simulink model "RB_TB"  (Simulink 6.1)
settings: Solver=ode3  SolverMode=SingleTasking  StartTime=0  StopTime=0.1  FixedStep=0.01  RelTol=1e-3
libraries: simulink x2
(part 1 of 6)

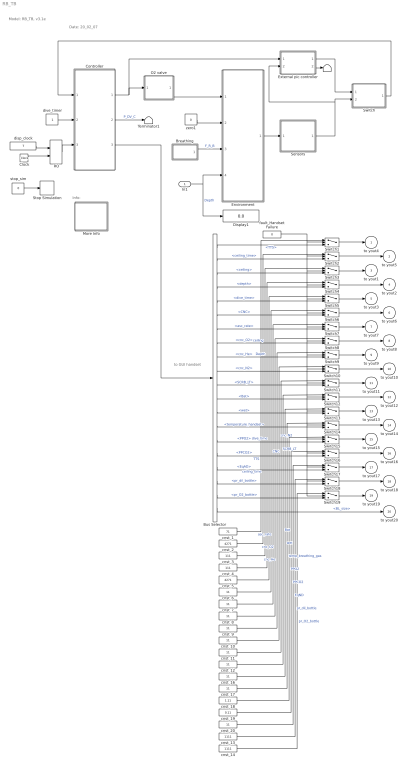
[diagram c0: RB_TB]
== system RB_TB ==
  note: Model: RB_TB, v3.1e
  note: Date: 20_02_07
  note: to GUI handset
  note: Info:
  In1 : Inport  Port=1  LatchInput=off
  Breathing : Subsystem
  Bus Selector : BusSelector  DialogController=Simulink.DDGSource_Bus  OutputSignals=TTS,ceiling_time,ceiling,depth,dive_time,CNC,asc_rate,cnc_O2,cnc_He,cnc_N2,SCRB_LT,Bat,wet,temperature_handset,PPO2,PPCO2,EqAD,pr_dil_bottle,pr_O2_bottle,BL_size
  Clock : Clock
  Controller : Subsystem
  Display1 : Display
  Environment : Subsystem
  External pic controller : Subsystem
  More Info : Subsystem
  O2 valve : Subsystem
  RO : RelationalOperator  Operator===  LogicOutDataTypeMode=Boolean
  Sensors : Subsystem
  Stop Simulation : Stop
  Switch : Subsystem
  Switch{1..19} (19 alike) : Switch  Threshold=0.5
  T : Terminator
  Terminator1 : Terminator
  cnst_1 : Constant  Value=71
  cnst_{6..12,16..17,20} (10 alike) : Constant  Value=11
  cnst_13 : Constant  Value=1111
  cnst_14 : Constant  Value=1111
  cnst_18 : Constant  Value=1.11
  cnst_19 : Constant  Value=0.11
  cnst_2 : Constant  Value=4271
  cnst_3 : Constant  Value=111
  cnst_4 : Constant  Value=111
  cnst_5 : Constant  Value=4271
  disp_clock : Constant  Value=7
  dive_timer : Constant
  fault_Handset Failure : Constant  Value=0
  stop_sim : Constant  Value=0
  zero1 : Constant  Value=0
  to yout4 : Outport
  to yout5 : Outport  Port=2
  to yout1 : Outport  Port=3
  to yout2 : Outport  Port=4
  to yout3 : Outport  Port=5
  to yout6 : Outport  Port=6
  to yout7 : Outport  Port=7
  to yout8 : Outport  Port=8
  to yout9 : Outport  Port=9
  to yout10 : Outport  Port=10
  to yout11 : Outport  Port=11
  to yout12 : Outport  Port=12
  to yout13 : Outport  Port=13
  to yout14 : Outport  Port=14
  to yout15 : Outport  Port=15
  to yout16 : Outport  Port=16
  to yout17 : Outport  Port=17
  to yout18 : Outport  Port=18
  to yout19 : Outport  Port=19
  to yout20 : Outport  Port=20
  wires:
  Controller/1(O2 control) -> O2 valve/1(IN), External pic controller/1(valve_in)
  Breathing/1(Metabolic) -> Environment/3(Metablic)  "F_R_B"
  Environment/1(bus) -> Sensors/1(In)
  disp_clock/1 -> RO/1
  Clock/1 -> RO/2
  RO/1 -> Controller/3(disp_clock)
  External pic controller/1(sensor_out) -> Switch/1(In1)
  Sensors/1(Out) -> Switch/2(In2), External pic controller/2(sensor_in)
  Switch/1(Out) -> Controller/1(InBus)
  Controller/2(Dil valve) -> Terminator1/1  "P_DV_C"
  zero1/1 -> Environment/2(Dil valve)
  O2 valve/1(Orf_size) -> Environment/1(Orf_size)
  dive_timer/1 -> Controller/2(dive_timer)
  cnst_1/1 -> Switch1/1  "TTS"
  cnst_2/1 -> Switch2/1  "ceiling_time"
  cnst_4/1 -> Switch4/1  "Depth"
  cnst_5/1 -> Switch5/1  "dive_time"
  cnst_6/1 -> Switch6/1  "CNC"
  cnst_7/1 -> Switch7/1  "asc_rate"
  cnst_8/1 -> Switch8/1  "cnc_O2"
  cnst_9/1 -> Switch9/1  "cnc_He"
  cnst_10/1 -> Switch10/1  "cnc_N2"
  cnst_11/1 -> Switch11/1  "SCRB_LT"
  cnst_12/1 -> Switch12/1  "Bat"
  cnst_16/1 -> Switch13/1  "wet"
  cnst_17/1 -> Switch14/1  "temp_breathing_gas"
  cnst_18/1 -> Switch15/1  "PPO2"
  cnst_19/1 -> Switch16/1  "PPCO2"
  cnst_20/1 -> Switch17/1  "EqND"
  cnst_13/1 -> Switch18/1  "pr_dil_bottle"
  cnst_14/1 -> Switch19/1  "pr_O2_bottle"
  Controller/3(bus) -> Bus Selector/1
  Bus Selector/1 -> Switch1/3  "<TTS>"
  Bus Selector/2 -> Switch2/3  "<ceiling_time>"
  Bus Selector/3 -> Switch3/3  "<ceiling>"
  Bus Selector/4 -> Switch4/3  "<depth>"
  Bus Selector/5 -> Switch5/3  "<dive_time>"
  Bus Selector/6 -> Switch6/3  "<CNC>"
  Bus Selector/7 -> Switch7/3  "<asc_rate>"
  Bus Selector/8 -> Switch8/3  "<cnc_O2>"
  Bus Selector/9 -> Switch9/3  "<cnc_He>"
  Bus Selector/10 -> Switch10/3  "<cnc_N2>"
  Bus Selector/11 -> Switch11/3  "<SCRB_LT>"
  Bus Selector/12 -> Switch12/3  "<Bat>"
  Bus Selector/13 -> Switch13/3  "<wet>"
  Bus Selector/14 -> Switch14/3  "<temperature_handset>"
  Bus Selector/15 -> Switch15/3  "<PPO2>"
  Bus Selector/16 -> Switch16/3  "<PPCO2>"
  Bus Selector/17 -> Switch17/3  "<EqAD>"
  Bus Selector/18 -> Switch18/3  "<pr_dil_bottle>"
  Bus Selector/19 -> Switch19/3  "<pr_O2_bottle>"
  Switch19/1 -> to yout19/1
  Switch18/1 -> to yout18/1
  Switch17/1 -> to yout17/1
  Switch16/1 -> to yout16/1
  Switch15/1 -> to yout15/1
  Switch14/1 -> to yout14/1
  Switch13/1 -> to yout13/1
  Switch12/1 -> to yout12/1
  Switch11/1 -> to yout11/1
  Switch10/1 -> to yout10/1
  Switch9/1 -> to yout9/1
  Switch8/1 -> to yout8/1
  Switch7/1 -> to yout7/1
  Switch6/1 -> to yout6/1
  Switch5/1 -> to yout3/1
  Switch4/1 -> to yout2/1
  Switch3/1 -> to yout1/1
  Switch2/1 -> to yout5/1
  Switch1/1 -> to yout4/1
  fault_Handset Failure/1 -> Switch18/2, Switch19/2, Switch17/2, Switch16/2, Switch15/2, Switch14/2, Switch13/2, Switch12/2, Switch11/2, Switch10/2, Switch9/2, Switch8/2, Switch7/2, Switch6/2, Switch5/2, Switch4/2, Switch3/2, Switch2/2, Switch1/2
  In1/1 -> Display1/1, Environment/4(Depth)  "Depth"
  External pic controller/2(valve_out) -> T/1
  cnst_3/1 -> Switch3/1  "ceiling"
  stop_sim/1 -> Stop Simulation/1
  Bus Selector/20 -> to yout20/1  "<BL_size>"

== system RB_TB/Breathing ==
  note: Model: RB_TB/Breathing
  rate_metabolic : Sin  Amplitude=0.015  Bias=0.015  Frequency=1.4661  SampleTime=0
  Metabolic : Outport
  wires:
  rate_metabolic/1 -> Metabolic/1

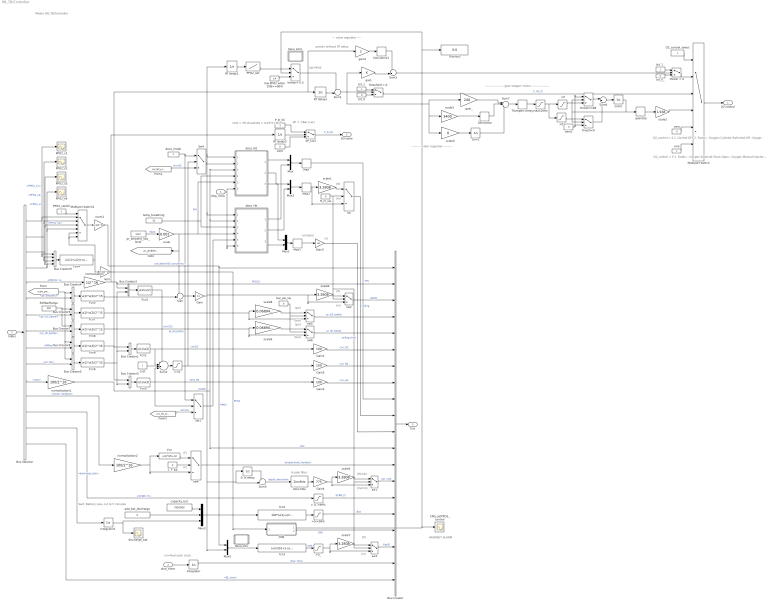
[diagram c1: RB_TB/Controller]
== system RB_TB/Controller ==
  note: Model: RB_TB/Controller
  note: dP = -1Bar (var)
  note: CO2 = 3% threshold = 0.03*2^16
  note: (minute)
  note: (s)
  note: ini=final each clock
  note: Fault: Battery Low, cut to 5 minutes
  note: predicr without RT delay
  note: O2_control = 4 1. Control OFF 2. Faults: - Oxygen Cylinder Switched Off - Oxygen First Stage Failure - Oxygen Solenoid Stuck Closed
  note: O2_control = 5 1. Faults: - Oxygen Solenoid Stuck Open - Oxygen Manual Injector Failure
  note: 6-pole filter
  note: ------------------- gear stepper motor ------------------
  note: Set PPO2
  note: --------- motor regulator ---------
  note: --- valve regulator ----
  note: (m)
  note: (ft)
  note: (ft)
  note: (m)
  note: (ft/min)
  note: (m/min)
  note: (m)
  note: (ft)
  note: (C)
  note: (F)
  note: (psi)
  note: (bar)
  note: (psi)
  note: (bar)
  note: HANDSET ALARM
  InBus : Inport  Port=1  LatchInput=off
  dive_timer : Inport  Port=2  LatchInput=off
  disp_clock : Inport  Port=3  LatchInput=off
  0.1s delay : UnitDelay  SampleTime=0.1
  300barRange : Constant  Value=300
  <0 : Saturate  UpperLimit=0  LowerLimit=-inf
  "> 0, <99%" : Saturate  UpperLimit=99  LowerLimit=0
  >0 : Saturate  UpperLimit=inf  LowerLimit=0
  >0,<99% : Saturate  UpperLimit=99  LowerLimit=0
  >0_ : Saturate  UpperLimit=inf  LowerLimit=0
  >=0 : Saturate  UpperLimit=inf  LowerLimit=0
  Bus Creator : BusCreator  DialogController=Simulink.DDGSource_Bus  Inputs=20
  Bus Creator{1..8} (8 alike) : BusCreator  DialogController=Simulink.DDGSource_Bus  Inputs=2
  Bus Creator9 : BusCreator  DialogController=Simulink.DDGSource_Bus
  Bus Selector : BusSelector  DialogController=Simulink.DDGSource_Bus  OutputSignals=PPO2_s1,PPO2_s2,PPO2_s3,PPO2_s4,PPCO2_s,pr_ambient,pr_O2_bottle,pr_dil_bottle,PPHe,pr_BL,wet,temp_handset,SCRB_LT,discharge_bat,BL_size
  CNS : Subsystem
  CNS_setPPO2_control : Scope
  C_F_sw : Constant  Value=0
  Derivative : Derivative
  Derivative1 : Derivative
  Display2 : Display
  Fcn : Fcn  Expr=u(1)*9/5+32
  Fcn1 : Fcn  Expr=u(1)/u(2)
  Fcn2 : Fcn  Expr=u(1)/u(2)
  Fcn3 : Fcn  Expr=u(1)/u(2)
  Fcn4 : Fcn  Expr=(u(1)+u(2)+u(3)+u(4))/4
  Fcn{5..8} (4 alike) : Fcn  Expr=u(1)*u(2)/2^15
  Fcn9 : Fcn  Expr=u(1)*u(2)/2^16
  Gain : Gain  Gain=10
  Gain1 : Gain  Gain=100
  Gain2 : Gain  Gain=100
  Gain3 : Gain  Gain=60
  Gain4 : Gain  Gain=775
  Gain5 : Gain  Gain=100
  Integrator : Integrator
  Integrator1 : Integrator
  Max : MinMax  Function=max
  Max1 : MinMax  Function=max
  Max2 : MinMax  Function=max
  More Info : Subsystem
  More Info1 : Subsystem
  Multiport Switch : MultiPortSwitch  Inputs=5
  Multiport Switch1 : MultiPortSwitch  Inputs=6
  Mux{,1..2,5} (4 alike) : Mux  Inputs=2
  Mux3 : Mux  Inputs=3
  O2_control_select : Constant
  PPO2_s{1..4} (4 alike) : Scope
  PPO2_set : Lookup  DialogController=Simulink.DDGSource  InputValues="[0         4.3001           1000]"  OutputValues="[0.7      1.0001      1.0002]"  LookUpMeth=Interpolation-Use End Values
  PPO2_switch : Constant
  P_D_VC : Constant  Value=-1
  RT delay1 : UnitDelay  SampleTime=0.1
  RT delay2 : UnitDelay  SampleTime=0.1
  RT delay3 : UnitDelay  SampleTime=0.1
  SP_CO2 : Switch  Threshold=0.03
  Sum : Sum  Inputs=-+|
  Sum1 : Sum  Inputs=+-|
  Sum2 : Sum  Inputs=--+-|
  Sum3 : Sum  Inputs=-+|
  Sum4 : Sum  Inputs=|++
  Sum5 : Sum  Inputs=-+|
  Sum7 : Sum  Inputs=|+++
  Sw1 : MultiPortSwitch  Inputs=2
  Sw4 : MultiPortSwitch  Inputs=2
  Transport Delay : TransportDelay  DelayTime=0.01
  Zero : Constant  Value=0
  Zero-Pole : ZeroPole  Zeros=[0]  Poles=[-1 -1 -1 -1 -1 -1]
  add_bat_discharge : Constant  Value=0
  bar_psi_sw : Constant  Value=0
  bit_0 : Constant  Value=0
  bit_0_ : Constant  Value=0
  bit_1 : Constant
  bit_1_ : Constant
  capacity_bat : Constant  Value=7920000
  cnst : Constant
  deco_He : Subsystem
  deco_N2 : Subsystem
  deco_mode : Constant
  discharge_bat : Scope
  fcn2 : Fcn  Expr=100*(u(1)-u(2)-u(3))/u(1)
  fcn3 : Fcn  Expr=(u(2)/10+1-u(1))/0.79-1
  ft_m_sw : Constant  Value=0
  gain : Gain
  gain1 : Gain  Gain=2
  gain_ : Gain  Gain=240
  low PPO2 when CNS>=90% : Constant  Value=0.4
  max100Hz : Saturate  UpperLimit=100  LowerLimit=-100
  norm : Gain  Gain=2.3/2^16
  norm1 : Gain  Gain=2.3/2^16
  normalisation : Gain  Gain=1/2^16
  normalisation1 : Gain  Gain=100/2^16
  normalisation2 : Gain  Gain=100/2^16
  one : Constant
  pr_ambient_sea_level : Constant  Value=1010
  quantize : Quantizer  QuantizationInterval=1
  scale : Gain  Gain=0.001
  scale{1,5..7} (4 alike) : Gain  Gain=3.2808
  scale2 : Gain  Gain=1/168
  scale3 : Gain  Gain=3400
  scale4 : Gain  Gain=0
  scale8 : Gain  Gain=0.0689476
  scale9 : Gain  Gain=0.0689476
  sum1 : Integrator
  sum2 : Integrator
  sw{,1..6} (7 alike) : Switch  Threshold=0.5
  temp_breathing : Constant  Value=33
  thresh = 0 : Switch  Criteria=u2 > Threshold
  thresh= 0.5 : Switch  Threshold=0.5
  thresh=0 : Switch
  thresh=168 : Switch  Threshold=168
  threshold = 0 : Switch  Criteria=u2 > Threshold
  zero : Constant  Value=0
  zero1 : Constant  Value=0
  O2 control : Outport
  Dil valve : Outport  Port=2
  bus : Outport  Port=3
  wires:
  RT delay2/1 -> Sum1/2
  bit_1/1 -> threshold = 0/1
  bit_0/1 -> threshold = 0/3
  temp_breathing/1 -> deco_N2/4(Temp_air), deco_He/3(Temp_air)
  deco_N2/1(TTS_N2) -> Mux/1
  deco_He/1(TTS_He) -> Mux/2
  Mux/1 -> Max/1
  Mux1/1 -> Max1/1
  deco_He/3(ceiling_time_He) -> Mux1/2
  deco_N2/3(ceiling_time_N2) -> Mux1/1
  Mux2/1 -> Max2/1
  deco_N2/2(ceiling_N2) -> Mux2/1
  deco_He/2(ceiling_He) -> Mux2/2
  Max/1 -> Bus Creator/9  "TTS"
  pr_ambient_sea_level/1 -> scale/1  "mbar"
  Bus Creator/1 -> bus/1
  InBus/1 -> Bus Selector/1
  Bus Selector/3 -> Bus Creator9/3, Multiport Switch1/4, PPO2_s3/1  "<PPO2_s3>"
  Bus Selector/4 -> Bus Creator9/4, Multiport Switch1/5, PPO2_s4/1  "<PPO2_s4>"
  norm/1 -> CNS/1(PPO2), RT delay2/1, gain1/1, Bus Creator1/1  "PPO2"
  normalisation/1 -> RT delay3/1, Bus Creator2/1, Bus Creator/2  "PPCO2"
  Sum/1 -> Gain/1
  Gain/1 -> 0.1s delay/1, Sum5/2, Mux5/2, deco_He/1(depth), deco_N2/1(depth), RT delay1/1, scale6/1, sw2/3  "Depth"
  Gain5/1 -> Bus Creator/7  "cnc_N2"
  Fcn3/1 -> Sum2/4, Sw1/2, Gain2/1  "sens He"
  disp_clock/1 -> deco_N2/6(disp_clock), deco_He/6(disp_clock)
  Integrator/1 -> Bus Creator/19  "dive_time"
  >0,<99%/1 -> Bus Creator/16  "Bat"
  RT delay3/1 -> SP_CO2/2
  P_D_VC/1 -> SP_CO2/1
  SP_CO2/1 -> Dil valve/1  "P_D_VC"
  Zero/1 -> SP_CO2/3
  Bus Selector/5 -> normalisation/1  "<PPCO2_s>"
  scale/1 -> deco_He/4(P_amb_sea_level), deco_N2/5(P_amb_sea_level), [pr_ambient_sea_level], Sum/1  "bar"
  Max1/1 -> Gain3/1
  Gain3/1 -> Bus Creator/11  "ceiling_time"
  Mux3/1 -> fcn2/1
  fcn2/1 -> >0,<99%/1
  Fcn1/1 -> Sum2/2, Gain1/1  "cncO2"
  Gain1/1 -> Bus Creator/6  "cnc_O2"
  Gain2/1 -> Bus Creator/8  "cnc_He"
  Bus Creator2/1 -> Fcn2/1
  cnst/1 -> Sum2/3
  Fcn2/1 -> Sum2/1  "cncCO2"
  deco_mode/1 -> Sw4/1, Sw1/1
  [cnc_N2_presize] -> Sw4/3  "sim N2"
  [cnc_He_presize] -> Sw1/3  "sim He"
  Sw4/1 -> deco_N2/2(cnc_N2)
  Sw1/1 -> deco_He/5(cnc_He)
  Mux5/1 -> fcn3/1
  fcn3/1 -> >0_/1  "CNS"
  CNS/2(CNS) -> Bus Creator/17  "CNC"
  dive_timer/1 -> Integrator/1
  capacity_bat/1 -> Mux3/1
  add_bat_discharge/1 -> Mux3/2
  Integrator1/1 -> discharge_bat/1, Mux3/3
  Bus Selector/2 -> Bus Creator9/2, Multiport Switch1/3, PPO2_s2/1  "<PPO2_s2>"
  Bus Selector/1 -> Multiport Switch1/2, Bus Creator9/1, PPO2_s1/1  "<PPO2_s1>"
  Sum1/1 -> gain/1, threshold = 0/2, gain_/1, scale4/1, scale3/1
  gain1/1 -> Derivative1/1
  O2_control_select/1 -> Multiport Switch/1
  Multiport Switch/1 -> O2 control/1
  bit_1_/1 -> thresh = 0/1
  bit_0_/1 -> thresh = 0/3
  Sum3/1 -> thresh = 0/2
  thresh = 0/1 -> Multiport Switch/2
  threshold = 0/1 -> Multiport Switch/3  "F_O2_O"
  "> 0, <99%"/1 -> Bus Creator/15  "SCRB_LT"
  Bus Selector/14 -> Integrator1/1  "<discharge_bat>"
  Bus Selector/13 -> "> 0, <99%"/1  "<SCRB_LT>"
  Bus Selector/11 -> normalisation1/1  "<wet>"
  normalisation1/1 -> deco_He/2(Wet), deco_N2/3(Wet), Bus Creator/12  "wet"
  Bus Selector/12 -> normalisation2/1  "<temp_handset>"
  [scale_pressure] -> Bus Creator4/1, Bus Creator5/1, Bus Creator8/1
  Bus Selector/6 -> Bus Creator4/2  "<pr_ambient>"
  Bus Creator4/1 -> Fcn5/1
  Fcn5/1 -> Sum/2
  Sum2/1 -> >=0/1
  >=0/1 -> Sw4/2, Gain5/1  "calculated N2 concentration"
  one/1 -> Multiport Switch/6
  Bus Creator3/1 -> Fcn3/1
  Bus Creator1/1 -> Fcn1/1
  Bus Creator5/1 -> Fcn6/1
  Bus Selector/10 -> Bus Creator5/2  "<pr_BL>"
  Fcn6/1 -> Bus Creator3/2, Bus Creator1/2, Bus Creator2/2
  Sum5/1 -> Zero-Pole/1  "depth_derivative"
  0.1s delay/1 -> Sum5/1
  Zero-Pole/1 -> Gain4/1
  Bus Selector/7 -> Bus Creator6/2  "<pr_O2_bottle>"
  Bus Creator6/1 -> Fcn7/1
  300barRange/1 -> Bus Creator6/1, Bus Creator7/1
  Bus Creator7/1 -> Fcn8/1
  Bus Selector/8 -> Bus Creator7/2  "<pr_dil_bottle>"
  Bus Creator8/1 -> Fcn9/1
  Bus Selector/9 -> Bus Creator8/2  "<PPHe>"
  Fcn9/1 -> Bus Creator3/1
  max100Hz/1 -> >0/1, <0/1
  Transport Delay/1 -> max100Hz/1
  scale3/1 -> Derivative/1
  scale4/1 -> sum1/1
  gain/1 -> Sum3/2
  Derivative1/1 -> Sum3/1
  scale2/1 -> Multiport Switch/4
  sum1/1 -> Sum7/3
  Max2/1 -> scale1/1, sw/3
  scale1/1 -> sw/1
  ft_m_sw/1 -> sw/2, sw2/2, sw1/2, sw3/2
  sw/1 -> Bus Creator/10  "ceiling"
  scale5/1 -> sw1/1
  sw1/1 -> Bus Creator/14  "asc_rate"
  Gain4/1 -> sw1/3, scale5/1
  scale6/1 -> sw2/1
  sw2/1 -> Bus Creator/3  "depth"
  sw3/1 -> Bus Creator/18  "EqAD"
  scale7/1 -> sw3/1
  >0_/1 -> sw3/3, scale7/1
  Fcn/1 -> sw4/1
  C_F_sw/1 -> sw4/2
  sw4/1 -> Bus Creator/13  "temperature_handset"
  normalisation2/1 -> sw4/3, Fcn/1
  Fcn7/1 -> scale8/1, sw5/3
  bar_psi_sw/1 -> sw5/2, sw6/2
  scale8/1 -> sw5/1
  sw5/1 -> Bus Creator/4  "pr_O2_bottle"
  Fcn8/1 -> sw6/3, scale9/1  "pr_dil_bottle"
  scale9/1 -> sw6/1
  sw6/1 -> Bus Creator/5  "pr_dil_bottle"
  PPO2_switch/1 -> Multiport Switch1/1
  RT delay1/1 -> PPO2_set/1
  low PPO2 when CNS>=90%/1 -> thresh= 0.5/3
  CNS/1(PPO2_set_Control) -> CNS_setPPO2_control/1, thresh= 0.5/2, Display2/1
  >0/1 -> thresh=168/3
  <0/1 -> thresh=0/1
  quantize/1 -> scale2/1
  zero/1 -> Multiport Switch/5
  Multiport Switch1/1 -> norm1/1
  norm1/1 -> Bus Creator/1, Mux5/1  "PPO2"
  Bus Creator9/1 -> Fcn4/1
  Fcn4/1 -> norm/1, Multiport Switch1/6, Multiport Switch1/7
  Derivative/1 -> Sum7/2
  Sum7/1 -> Transport Delay/1
  gain_/1 -> Sum7/1
  sum2/1 -> quantize/1, thresh=168/2, thresh=0/2
  thresh=168/1 -> Sum4/1
  Sum4/1 -> sum2/1
  thresh=0/1 -> Sum4/2
  zero1/1 -> thresh=0/3, thresh=168/1
  Bus Selector/15 -> Bus Creator/20  "<BL_size>"
  PPO2_set/1 -> thresh= 0.5/1
  thresh= 0.5/1 -> Sum1/1

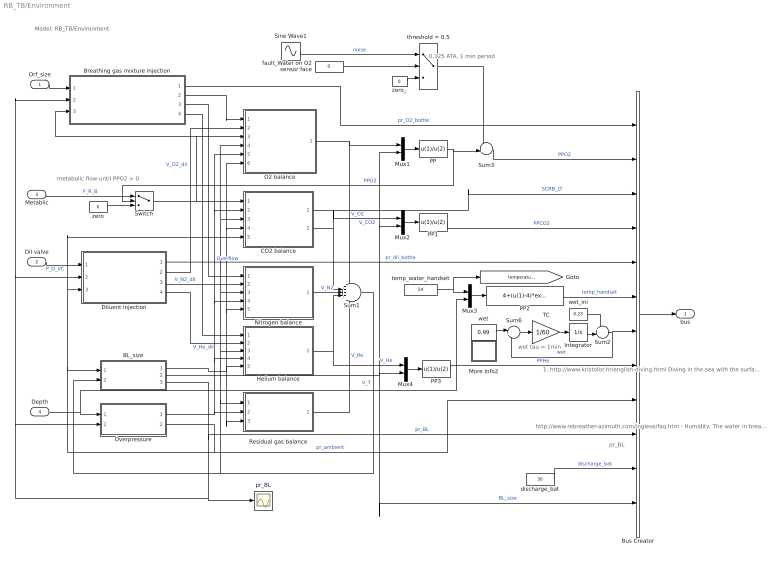
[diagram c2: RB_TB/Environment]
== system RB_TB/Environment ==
  note: Model: RB_TB/Environment
  note: metabolic flow until PPO2 > 0
  note: 0.125 ATA, 1 min period
  note: 1. http://www.kristofor.hr/english-diving.html Diving in the sea with the surface sea temperature 9 - 12 deg.C in winter, 24 - 28 degC in summer, On 20 m sea depth temperature is permanent, around 14 deg.C temperature = 14+(u(1)-14)*exp(-u(2)/7) 2. Al: Temperature goes from whatever the surface is, to 4C at 200m, and stays there below 200m. temperature = 4+(u(1)-4)*exp(-u(2)/35)
  note: http://www.rebreather-azimuth.com/inglese/faq.htm - Humidity: The water in breathing and from the chemical reaction maintain the humidity constantly at 100% in in semiclosed rebreather. The situation in open circuit is different, the gas mixture is completely dry, and the diver loses a big quantity of liquids during the dive.
  note: wet tau = 1min
  note: pr_BL
  Orf_size : Inport  Port=1  LatchInput=off
  Dil valve : Inport  Port=2  LatchInput=off
  Metablic : Inport  Port=3  LatchInput=off
  Depth : Inport  Port=4  LatchInput=off
  BL_size : Subsystem
  Breathing gas mixture injection : Subsystem
  Bus Creator : BusCreator  DialogController=Simulink.DDGSource_Bus  Inputs=12
  CO2 balance : Subsystem
  Diluent injection : Subsystem
  Helium balance : Subsystem
  Integrator : Integrator
  More Info2 : Subsystem
  Mux{1..4} (4 alike) : Mux  Inputs=2
  Nitrogen balance : Subsystem
  O2 balance : Subsystem
  Overpressure : Subsystem
  PP : Fcn  Tag=ee  Priority=306454640  Expr=u(1)/u(2)
  PP1 : Fcn  Tag=ee  Priority=306454640  Expr=u(1)/u(2)
  PP2 : Fcn  Tag=ee  Priority=306454640  Expr=4+(u(1)-4)*exp(-u(2)/35)
  PP3 : Fcn  Tag=ee  Priority=306454640  Expr=u(1)/u(2)
  Residual gas balance : Subsystem
  Sine Wave1 : Sin  Amplitude=0.125  Frequency=pi/30  SampleTime=0
  Sum1 : Sum  Inputs=+++++
  Sum2 : Sum  Inputs=++|
  Sum3 : Sum  Inputs=++|
  Sum6 : Sum  Inputs=|+-
  Switch : Switch  Criteria=u2 > Threshold
  TC : Gain  Gain=1/60
  discharge_bat : Constant  Value=30
  fault_Water on O2 sensor face : Constant  Value=0
  pr_BL : Scope
  temp_water_handset : Constant  Value=24
  threshold = 0.5 : Switch  Criteria=u2 > Threshold  Threshold=0.5
  wet : Constant  Value=0.99
  wet_ini : Constant  Value=0.23
  zero : Constant  Value=0
  zero_ : Constant  Value=0
  bus : Outport
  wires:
  Diluent injection/3(N2) -> Nitrogen balance/2(V_N2_dil)  "V_N2_dil"
  O2 balance/1(O2 in BL) -> Sum1/1, Mux1/1  "V_O2"
  Overpressure/1(Overflow) -> CO2 balance/2(Overflow), O2 balance/5(Overflow), Nitrogen balance/4(Overflow), Helium balance/4(Overflow), Residual gas balance/2(Overflow)  "Overflow"
  Sum1/1 -> Helium balance/3(gas_total), Nitrogen balance/3(gas_total), CO2 balance/3(gas_total), O2 balance/4(gas_total), Residual gas balance/1(gas_total), BL_size/2(vol_gas_total)  "V_T"
  Nitrogen balance/1(N2 in BL) -> Sum1/3  "V_N2"
  CO2 balance/2(CO2 in BL) -> Sum1/2, Mux2/1  "V_CO2"
  Dil valve/1 -> Diluent injection/1(Valve_ON/OFF)  "P_D_VC"
  Helium balance/1(He in BL) -> Mux4/1, Sum1/4  "V_He"
  Diluent injection/4(He) -> Helium balance/2(V_He_dil)  "V_He_dil"
  Residual gas balance/1(Re in BL) -> Sum1/5  "V_Re"
  PP/1 -> Sum3/2, Switch/2  "PPO2"
  Bus Creator/1 -> bus/1
  PP1/1 -> Bus Creator/4  "PPCO2"
  PP3/1 -> Bus Creator/8  "PPHe"
  BL_size/2(BL_size) -> Mux4/2, Mux2/2, Mux1/2, Bus Creator/12  "BL_size"
  Mux1/1 -> PP/1
  Mux2/1 -> PP1/1
  Mux4/1 -> PP3/1
  Orf_size/1 -> Breathing gas mixture injection/1(Orf_size)
  Breathing gas mixture injection/1(pr_breathing_mixture_bottle) -> Bus Creator/1  "pr_O2_bottle"
  Overpressure/2(pr_ambient) -> Bus Creator/9, BL_size/1(pr_ambient), Diluent injection/3(pr_ambient), CO2 balance/5(pr_ambient)  "pr_ambient"
  Diluent injection/1(pr_dil_bottle) -> Bus Creator/5  "pr_dil_bottle"
  BL_size/3(pr_BL) -> Overpressure/2(pr_BL), Breathing gas mixture injection/2(pr_BL), Diluent injection/2(pr_BL), pr_BL/1, Bus Creator/10  "pr_BL"
  Depth/1 -> Overpressure/1(Depth), Mux3/2
  Switch/1 -> CO2 balance/1(Metabolic), O2 balance/3(Metabolic), Breathing gas mixture injection/3(Metabolic)
  Metablic/1 -> Switch/1  "F_R_B"
  zero/1 -> Switch/3
  CO2 balance/1(SCRB) -> Bus Creator/3  "SCRB_LT"
  discharge_bat/1 -> Bus Creator/11  "discharge_bat"
  fault_Water on O2 sensor face/1 -> threshold = 0.5/2
  Sine Wave1/1 -> threshold = 0.5/1  "noise"
  zero_/1 -> threshold = 0.5/3
  Sum3/1 -> Bus Creator/2  "PPO2"
  threshold = 0.5/1 -> Sum3/1
  temp_water_handset/1 -> Mux3/1, [temperature_sea_level]
  Mux3/1 -> PP2/1
  PP2/1 -> Bus Creator/6  "temp_handset"
  TC/1 -> Integrator/1
  Integrator/1 -> Sum2/2
  wet_ini/1 -> Sum2/1
  Sum2/1 -> Sum6/2, Bus Creator/7  "wet"
  Sum6/1 -> TC/1
  wet/1 -> Sum6/1
  Diluent injection/2(O2) -> O2 balance/2(V_O2_dil)  "V_O2_dil"
  Breathing gas mixture injection/2(V_O2_breathing_mixture_bottle) -> O2 balance/1(V_O2_breathing)
  Breathing gas mixture injection/3(V_N2_breathing_mixture_bottle) -> Nitrogen balance/1(V_N2_breathing)
  Breathing gas mixture injection/4(V_He_breathing_mixture_bottle) -> Helium balance/1(V_He_breathing)
  BL_size/1(BL_size_ini) -> Helium balance/5(BL_size_ini), Residual gas balance/3(BL_size_ini), Nitrogen balance/5(BL_size_ini), CO2 balance/4(BL_size_ini), O2 balance/6(BL_size_ini)

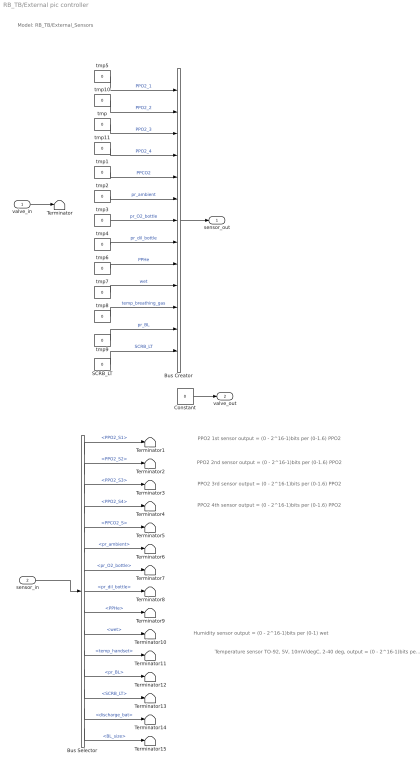
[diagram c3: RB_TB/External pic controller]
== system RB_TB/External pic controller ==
  note: Model: RB_TB/External_Sensors
  note: Humidity sensor output = (0 - 2^16-1)bits per (0-1) wet
  note: PPO2 1st sensor output = (0 - 2^16-1)bits per (0-1.6) PPO2
  note: PPO2 2nd sensor output = (0 - 2^16-1)bits per (0-1.6) PPO2
  note: PPO2 3rd sensor output = (0 - 2^16-1)bits per (0-1.6) PPO2
  note: PPO2 4th sensor output = (0 - 2^16-1)bits per (0-1.6) PPO2
  note: Temperature sensor TO-92, 5V, 10mV/degC, 2-40 deg, output = (0 - 2^16-1)bits per (0-1) wet
  valve_in : Inport  Port=1  LatchInput=off
  sensor_in : Inport  Port=2  LatchInput=off
  Bus Creator : BusCreator  DialogController=Simulink.DDGSource_Bus  Inputs=13
  Bus Selector : BusSelector  DialogController=Simulink.DDGSource_Bus  OutputSignals=PPO2_S1,PPO2_S2,PPO2_S3,PPO2_S4,PPCO2_S,pr_ambient,pr_O2_bottle,pr_dil_bottle,PPHe,wet,temp_handset,pr_BL,SCRB_LT,discharge_bat,BL_size
  Constant : Constant  Value=0
  SCRB_LT : Constant  Value=0
  Terminator{,1..15} (16 alike) : Terminator
  tmp{,1..11} (12 alike) : Constant  Value=0
  sensor_out : Outport
  valve_out : Outport  Port=2
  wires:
  tmp7/1 -> Bus Creator/10  "wet"
  tmp8/1 -> Bus Creator/11  "temp_breathing_gas"
  tmp6/1 -> Bus Creator/9  "PPHe"
  tmp4/1 -> Bus Creator/8  "pr_dil_bottle"
  tmp3/1 -> Bus Creator/7  "pr_O2_bottle"
  tmp2/1 -> Bus Creator/6  "pr_ambient"
  tmp1/1 -> Bus Creator/5  "PPCO2"
  Bus Creator/1 -> sensor_out/1
  tmp/1 -> Bus Creator/3  "PPO2_3"
  valve_in/1 -> Terminator/1
  tmp9/1 -> Bus Creator/12  "pr_BL"
  SCRB_LT/1 -> Bus Creator/13  "SCRB_LT"
  tmp5/1 -> Bus Creator/1  "PPO2_1"
  tmp10/1 -> Bus Creator/2  "PPO2_2"
  sensor_in/1 -> Bus Selector/1
  tmp11/1 -> Bus Creator/4  "PPO2_4"
  Bus Selector/1 -> Terminator1/1  "<PPO2_S1>"
  Bus Selector/2 -> Terminator2/1  "<PPO2_S2>"
  Bus Selector/3 -> Terminator3/1  "<PPO2_S3>"
  Bus Selector/4 -> Terminator4/1  "<PPO2_S4>"
  Bus Selector/5 -> Terminator5/1  "<PPCO2_S>"
  Bus Selector/9 -> Terminator9/1  "<PPHe>"
  Bus Selector/6 -> Terminator6/1  "<pr_ambient>"
  Bus Selector/7 -> Terminator7/1  "<pr_O2_bottle>"
  Bus Selector/8 -> Terminator8/1  "<pr_dil_bottle>"
  Bus Selector/10 -> Terminator10/1  "<wet>"
  Bus Selector/11 -> Terminator11/1  "<temp_handset>"
  Bus Selector/12 -> Terminator12/1  "<pr_BL>"
  Bus Selector/13 -> Terminator13/1  "<SCRB_LT>"
  Bus Selector/14 -> Terminator14/1  "<discharge_bat>"
  Constant/1 -> valve_out/1
  Bus Selector/15 -> Terminator15/1  "<BL_size>"

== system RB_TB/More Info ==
  note: The S-Function "depth_data" runs depth_data.m in real-time that calculates the current depth using the Depth table data. The Simulink subsytems are Valve controller and Breathing loop. Gas balance includes O2, CO2, N2, He and Reminder gas the O2 pressure reduction valve is not compensated to ambient pressure Controller includes: Bang-Bang O2 and CO2 control; calc of decompression The depth profile is profile.time = [time1, time2,..., timen], and profile.rate = [depth_ini, rate1, rate2,...raten ] 1b deco compartments for N2 and He are installed "a", "b" and Half-Time deco for H2 is updated tissue compartment of 1b deco for N2 and He are add the half_times of He are updated satuation of the PPO2 sensor is 1.6 round of the deco d_min is changed by ceil ceil of the deco ceiling time and asc_time is removed models of the SCRB, BAT, CNS and EqND parameters are installed
  note: The run file is main_RB_TB.m
  note: Temporary actions: 1) The 0.1s delay of PPO2 sensor is removed
  note: This system models the Re-Breather Test Bench. It includs analogue and digital parts. The revision history is in Readme.doc file
  note: PPCO2 controls is off

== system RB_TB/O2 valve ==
  note: Model: RB_TB/O2 valve
  IN : Inport  Port=1  LatchInput=off
  DAC 1bit : DataTypeConversion  OutDataTypeMode=double  ConvertRealWorld=Stored Integer (SI)  RndMeth=Nearest
  Orf_size : Outport
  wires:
  IN/1 -> DAC 1bit/1
  DAC 1bit/1 -> Orf_size/1

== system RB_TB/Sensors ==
  note: Model: RB_TB/Sensors
  note: Info:
  note: 10 mV corresponds to PPO2 of 0.2095 ATA 109.8 mV to 2.3 ATA 5 mV to 0.1048 ATA 20 mV to 0.419 ATA
  note: 10 mV corresponds to 5968 of 16bit ADC with saturation of 2.3 PPO2 109.8 mV to 65536 5 mV to 2984 20 mV to 11936
  note: Initial time constant of PPO2 sensors are 1.5; 1.75, 2, 2.5 s
  In : Inport  Port=1  LatchInput=off
  Bus Creator : BusCreator  DialogController=Simulink.DDGSource_Bus  Inputs=15
  Bus Selector : BusSelector  DialogController=Simulink.DDGSource_Bus  OutputSignals=PPO2,PPCO2,pr_ambient,pr_O2_bottle,pr_dil_bottle,PPHe,wet,temp_handset,pr_BL,SCRB_LT,discharge_bat,BL_size
  Humidity Sensor : Subsystem
  More Info : Subsystem
  PPCO2 sensor : Subsystem
  PPHe sensor : Subsystem
  PPO2 sensor1 : Subsystem
  PPO2 sensor2 : Subsystem
  PPO2 sensor3 : Subsystem
  PPO2 sensor4 : Subsystem
  PPO2_1_state : Constant  Value=0
  PPO2_2_state : Constant  Value=0
  PPO2_3_state : Constant  Value=0
  PPO2_4_state : Constant  Value=0
  Pressure_Br_Loop Sensor : Subsystem
  Pressure_O2_bottle_Sensor : Subsystem
  Pressure_ambient Sensor : Subsystem
  Pressure_dil_bottle_Sensor : Subsystem
  Temperature Sensor : Subsystem
  output_PPO2_{1..4} (4 alike) : Constant  Value=11936
  thresh = 0.1 : Switch  Criteria=u2 > Threshold  Threshold=0.5
  threshold = 0.3 : Switch  Criteria=u2 > Threshold  Threshold=0.5
  threshold = 0.5 : Switch  Criteria=u2 > Threshold  Threshold=0.5
  threshold = 0.5_1 : Switch  Criteria=u2 > Threshold  Threshold=0.5
  Out : Outport
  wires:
  In/1 -> Bus Selector/1
  Bus Creator/1 -> Out/1
  Bus Selector/1 -> PPO2 sensor3/1(PPO2), PPO2 sensor1/1(PPO2), PPO2 sensor2/1(PPO2), PPO2 sensor4/1(PPO2)  "<PPO2>"
  Bus Selector/2 -> PPCO2 sensor/1(PPCO2)  "<PPCO2>"
  PPCO2 sensor/1(PPCO2_S) -> Bus Creator/5  "PPCO2_S"
  Bus Selector/10 -> Bus Creator/13  "<SCRB_LT>"
  Bus Selector/11 -> Bus Creator/14  "<discharge_bat>"
  PPO2_1_state/1 -> threshold = 0.5/2
  output_PPO2_1/1 -> threshold = 0.5/1
  threshold = 0.3/1 -> Bus Creator/4  "PPO2_S4"
  Bus Selector/7 -> Humidity Sensor/1(in)  "<wet>"
  Humidity Sensor/1(out) -> Bus Creator/10  "wet"
  Bus Selector/8 -> Temperature Sensor/1(in)  "<temp_handset>"
  Temperature Sensor/1(out) -> Bus Creator/11  "temp_handset"
  Bus Selector/3 -> Pressure_ambient Sensor/1(in)  "<pr_ambient>"
  Pressure_ambient Sensor/1(out) -> Bus Creator/6  "pr_ambient"
  Bus Selector/9 -> Pressure_Br_Loop Sensor/1(in)  "<pr_BL>"
  Pressure_Br_Loop Sensor/1(out) -> Bus Creator/12  "pr_BL"
  Bus Selector/5 -> Pressure_dil_bottle_Sensor/1(in)  "<pr_dil_bottle>"
  Pressure_dil_bottle_Sensor/1(out) -> Bus Creator/8  "pr_dil_bottle"
  Bus Selector/4 -> Pressure_O2_bottle_Sensor/1(in)  "<pr_O2_bottle>"
  Pressure_O2_bottle_Sensor/1(out) -> Bus Creator/7  "pr_O2_bottle"
  PPHe sensor/1(PPHe_S) -> Bus Creator/9  "PPHe"
  Bus Selector/6 -> PPHe sensor/1(PPHe)  "<PPHe>"
  PPO2 sensor1/1(PPO2_S) -> threshold = 0.5/3
  PPO2_2_state/1 -> threshold = 0.5_1/2
  output_PPO2_2/1 -> threshold = 0.5_1/1
  PPO2 sensor2/1(PPO2_S) -> threshold = 0.5_1/3
  PPO2_3_state/1 -> thresh = 0.1/2
  output_PPO2_3/1 -> thresh = 0.1/1
  PPO2 sensor3/1(PPO2_S) -> thresh = 0.1/3
  PPO2_4_state/1 -> threshold = 0.3/2
  output_PPO2_4/1 -> threshold = 0.3/1
  PPO2 sensor4/1(PPO2_S) -> threshold = 0.3/3
  thresh = 0.1/1 -> Bus Creator/3  "PPO2_S3"
  threshold = 0.5_1/1 -> Bus Creator/2  "PPO2_S2"
  threshold = 0.5/1 -> Bus Creator/1  "PPO2_S1"
  Bus Selector/12 -> Bus Creator/15  "<BL_size>"

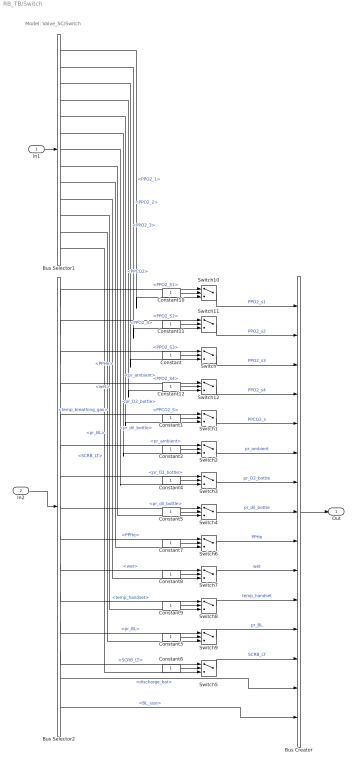
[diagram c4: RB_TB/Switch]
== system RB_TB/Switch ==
  note: Model: Valve_SC/Switch
  In1 : Inport  Port=1  LatchInput=off
  In2 : Inport  Port=2  LatchInput=off
  Bus Creator : BusCreator  DialogController=Simulink.DDGSource_Bus  Inputs=15
  Bus Selector1 : BusSelector  DialogController=Simulink.DDGSource_Bus  OutputSignals=PPO2_1,PPO2_2,PPO2_3,PPO2_4,PPCO2,pr_ambient,pr_O2_bottle,pr_dil_bottle,PPHe,wet,temp_breathing_gas,pr_BL,SCRB_LT
  Bus Selector2 : BusSelector  DialogController=Simulink.DDGSource_Bus  OutputSignals=PPO2_S1,PPO2_S2,PPO2_S3,PPO2_S4,PPCO2_S,pr_ambient,pr_O2_bottle,pr_dil_bottle,PPHe,wet,temp_handset,pr_BL,SCRB_LT,discharge_bat,BL_size
  Constant{,1..12} (13 alike) : Constant
  Switch{,1..12} (13 alike) : Switch
  Out : Outport
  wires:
  Switch7/1 -> Bus Creator/10  "wet"
  Switch8/1 -> Bus Creator/11  "temp_handset"
  Switch6/1 -> Bus Creator/9  "PPHe"
  Switch4/1 -> Bus Creator/8  "pr_dil_bottle"
  Switch3/1 -> Bus Creator/7  "pr_O2_bottle"
  Switch2/1 -> Bus Creator/6  "pr_ambient"
  Switch1/1 -> Bus Creator/5  "PPCO2_s"
  Switch/1 -> Bus Creator/3  "PPO2_s3"
  Bus Creator/1 -> Out/1
  Bus Selector1/7 -> Switch3/3  "<pr_O2_bottle>"
  In1/1 -> Bus Selector1/1
  Bus Selector1/6 -> Switch2/3  "<pr_ambient>"
  Bus Selector1/5 -> Switch1/3  "<PPCO2>"
  Bus Selector1/4 -> Switch12/3  "<PPO2_4>"
  Bus Selector1/3 -> Switch/3  "<PPO2_3>"
  Bus Selector2/8 -> Switch4/1  "<pr_dil_bottle>"
  In2/1 -> Bus Selector2/1
  Bus Selector2/7 -> Switch3/1  "<pr_O2_bottle>"
  Bus Selector2/6 -> Switch2/1  "<pr_ambient>"
  Bus Selector2/5 -> Switch1/1  "<PPCO2_S>"
  Constant/1 -> Switch/2
  Constant1/1 -> Switch1/2
  Constant2/1 -> Switch2/2
  Constant4/1 -> Switch3/2
  Constant5/1 -> Switch4/2
  Constant7/1 -> Switch6/2
  Constant8/1 -> Switch7/2
  Constant9/1 -> Switch8/2
  Bus Selector2/12 -> Switch9/1  "<pr_BL>"
  Constant3/1 -> Switch9/2
  Switch9/1 -> Bus Creator/12  "pr_BL"
  Bus Selector2/9 -> Switch6/1  "<PPHe>"
  Bus Selector2/10 -> Switch7/1  "<wet>"
  Bus Selector2/11 -> Switch8/1  "<temp_handset>"
  Bus Selector1/8 -> Switch4/3  "<pr_dil_bottle>"
  Bus Selector1/9 -> Switch6/3  "<PPHe>"
  Bus Selector1/10 -> Switch7/3  "<wet>"
  Bus Selector1/11 -> Switch8/3  "<temp_breathing_gas>"
  Bus Selector2/13 -> Switch5/1  "<SCRB_LT>"
  Constant6/1 -> Switch5/2
  Switch5/1 -> Bus Creator/13  "SCRB_LT"
  Bus Selector1/12 -> Switch9/3  "<pr_BL>"
  Bus Selector2/14 -> Bus Creator/14  "<discharge_bat>"
  Constant10/1 -> Switch10/2
  Constant11/1 -> Switch11/2
  Switch11/1 -> Bus Creator/2  "PPO2_s2"
  Switch10/1 -> Bus Creator/1  "PPO2_s1"
  Bus Selector2/3 -> Switch/1  "<PPO2_S3>"
  Bus Selector2/2 -> Switch11/1  "<PPO2_S2>"
  Bus Selector2/1 -> Switch10/1  "<PPO2_S1>"
  Bus Selector1/2 -> Switch11/3  "<PPO2_2>"
  Bus Selector1/1 -> Switch10/3  "<PPO2_1>"
  Bus Selector2/4 -> Switch12/1  "<PPO2_S4>"
  Constant12/1 -> Switch12/2
  Switch12/1 -> Bus Creator/4  "PPO2_s4"
  Bus Selector1/13 -> Switch5/3  "<SCRB_LT>"
  Bus Selector2/15 -> Bus Creator/15  "<BL_size>"

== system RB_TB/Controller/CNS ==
  note: Model: RB_TB/Controller/CNS
  note: a half-time of 90 minutes
  note: disconnects the integrator when CNS >= 100%
  note: mode offset
  PPO2 : Inport  Port=1  LatchInput=off
  100% : Switch  Threshold=100
  <=100% : Saturate  UpperLimit=100  LowerLimit=0
  CNS_2001 : Lookup  DialogController=Simulink.DDGSource  InputValues="[0  0.49999   0.5   0.6   0.7   0.8   0.9   1.0   1.1   1.2   1.25  1.3  1.35 1.4  1.45 1.5  1.55    1.6  1.66 2.4]"  OutputValues="[0   0  1/540 1/432 1/342 1/270 1/216 1/180 1/144 1/126 1/117 1/108 1/99 1/90 1/81 1/72 10/495  1/27 100 100]"  LookUpMeth=Interpolation-Use End Values
  CNS_mode : Constant  Value=0
  Gain : Gain  Gain=1.2836e-004
  Integrator : Integrator
  More Info2 : Subsystem
  Relay_90/85% : Relay  OnSwitchValue=90  OffSwitchValue=85  OnOutputValue=0  OffOutputValue=1
  Sum : Sum  Inputs=|+-
  Sum1 : Sum  Inputs=++|
  Switch1 : Switch  Threshold=0.5
  Th_0.5 : Switch  Threshold=0.5
  add_PPO2 : Constant  Value=0.3
  zero : Constant  Value=0
  zero1 : Constant  Value=0
  zero2 : Constant
  PPO2_set_Control : Outport
  CNS : Outport  Port=2
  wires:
  Switch1/1 -> Integrator/1
  Integrator/1 -> <=100%/1, Sum/2
  PPO2/1 -> Switch1/2, Sum1/2
  <=100%/1 -> CNS/1, 100%/2, Relay_90/85%/1
  zero/1 -> Sum/1
  Sum/1 -> Gain/1
  Gain/1 -> Switch1/3
  100%/1 -> Switch1/1
  CNS_2001/1 -> 100%/3
  zero1/1 -> 100%/1
  Sum1/1 -> CNS_2001/1
  add_PPO2/1 -> Sum1/1
  Th_0.5/1 -> PPO2_set_Control/1
  CNS_mode/1 -> Th_0.5/2
  zero2/1 -> Th_0.5/3
  Relay_90/85%/1 -> Th_0.5/1

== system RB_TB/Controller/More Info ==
  note: EqAD (Equivalent Air Depth)
  note: EADInBar = ( DepthInBar + 1 - PO2 ) / 0.79 -1, where 0.79 is fraction of N2 in air

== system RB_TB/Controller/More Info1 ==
  note: Sensor fusion by using a sliding observer for an underwater breathing system Salvatore Carotenuto, Luigi Iannelli, Sabato Manfredi, Stefania Santini e-mail: luigi.iannelli@unisannio.it, {salcarot, smanfred, stsantin}@unina.it ... The actual oxygen content in the breathed mixture must be within specific limits by considering that (i) the oxygen partial pressure inside the breathing loop should never fall below 0.16 [atm] to avoid hypoxia (it can rapidly bring the diver to unconsciousness [1]); (ii) breathing oxygen at high partial pressure (greater than 0.5 [atm]) can be toxic [2] (Central Nervous System (CNS) oxygen toxicity is related to both oxygen pressure level and duration of the exposure [3]).

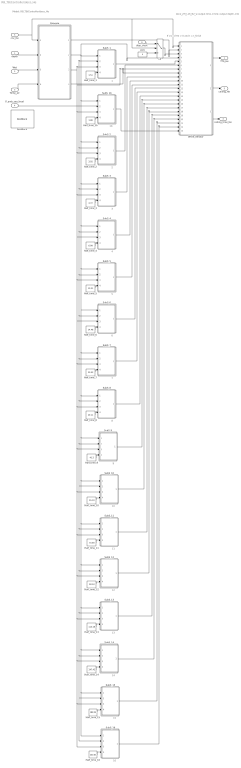
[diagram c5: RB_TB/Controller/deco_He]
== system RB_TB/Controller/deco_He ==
  note: 16
  note: 15
  note: 14
  note: 13
  note: 12
  note: 11
  note: 10
  note: 9
  note: 8
  note: 7
  note: 6
  note: 5
  note: 4
  note: 3
  note: 2
  note: 1
  note: deco_ZH_L16_N2_w output time, [min]; output depth, [m]
  note: Model: RB_TB/Controller/deco_He
  note: If cnc of He > 0 and t = t_finish
  note: 1b
  depth : Inport  Port=1  LatchInput=off
  Wet : Inport  Port=2  LatchInput=off
  Temp_air : Inport  Port=3  LatchInput=off
  P_amb_sea_level : Inport  Port=4  LatchInput=off
  cnc_He : Inport  Port=5  LatchInput=off
  disp_clock : Inport  Port=6  LatchInput=off
  >0 : Switch  Criteria=u2 > Threshold
  DocBlock : simulink/Model-Wide Utilities/DocBlock  DocumentType=Text
  Half_time_1 : Constant  Value=1.51
  Half_time_10 : Constant  Value=55.19
  Half_time_11 : Constant  Value=70.69
  Half_time_12 : Constant  Value=90.34
  Half_time_13 : Constant  Value=115.29
  Half_time_14 : Constant  Value=147.42
  Half_time_15 : Constant  Value=188.24
  Half_time_16 : Constant  Value=240.03
  Half_time_1b : Constant  Value=1.88
  Half_time_2 : Constant  Value=3.02
  Half_time_3 : Constant  Value=4.72
  Half_time_4 : Constant  Value=6.99
  Half_time_5 : Constant  Value=10.21
  Half_time_6 : Constant  Value=14.48
  Half_time_7 : Constant  Value=20.53
  Half_time_8 : Constant  Value=29.11
  Half_time_9 : Constant  Value=41.2
  Palveola : Subsystem
  SubS_1 : Subsystem
  SubS_10 : Subsystem
  SubS_11 : Subsystem
  SubS_12 : Subsystem
  SubS_13 : Subsystem
  SubS_14 : Subsystem
  SubS_15 : Subsystem
  SubS_16 : Subsystem
  SubS_1b : Subsystem
  SubS_2 : Subsystem
  SubS_3 : Subsystem
  SubS_4 : Subsystem
  SubS_5 : Subsystem
  SubS_6 : Subsystem
  SubS_7 : Subsystem
  SubS_8 : Subsystem
  SubS_9 : Subsystem
  While_Iterator : Subsystem  TreatAsAtomicUnit=on
  zero : Constant  Value=0
  TTS_He : Outport
  ceiling_He : Outport  Port=2
  ceiling_time_He : Outport  Port=3
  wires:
  Half_time_16/1 -> SubS_16/4(HT)
  Half_time_15/1 -> SubS_15/4(HT)
  Half_time_14/1 -> SubS_14/4(HT)
  Half_time_13/1 -> SubS_13/4(HT)
  Half_time_12/1 -> SubS_12/4(HT)
  Half_time_11/1 -> SubS_11/4(HT)
  Half_time_10/1 -> SubS_10/4(HT)
  Half_time_9/1 -> SubS_9/4(HT)
  Half_time_8/1 -> SubS_8/4(HT)
  Half_time_7/1 -> SubS_7/4(HT)
  Half_time_6/1 -> SubS_6/4(HT)
  Half_time_5/1 -> SubS_5/4(HT)
  Half_time_4/1 -> SubS_4/4(HT)
  Half_time_3/1 -> SubS_3/4(HT)
  Half_time_2/1 -> SubS_2/4(HT)
  Half_time_1/1 -> SubS_1/4(HT)
  SubS_16/1(bus) -> While_Iterator/22(In16)
  SubS_15/1(bus) -> While_Iterator/21(In15)
  SubS_14/1(bus) -> While_Iterator/20(In14)
  SubS_13/1(bus) -> While_Iterator/19(In13)
  SubS_12/1(bus) -> While_Iterator/18(In12)
  SubS_11/1(bus) -> While_Iterator/17(In11)
  SubS_10/1(bus) -> While_Iterator/16(In10)
  SubS_9/1(bus) -> While_Iterator/15(In9)
  SubS_8/1(bus) -> While_Iterator/14(In8)
  SubS_7/1(bus) -> While_Iterator/13(In7)
  SubS_6/1(bus) -> While_Iterator/12(In6)
  SubS_5/1(bus) -> While_Iterator/11(In5)
  SubS_4/1(bus) -> While_Iterator/10(In4)
  SubS_3/1(bus) -> While_Iterator/9(In3)
  Temp_air/1 -> Palveola/4(Temperature)
  Wet/1 -> Palveola/3(Humidity)
  While_Iterator/3(ceiling_time) -> ceiling_time_He/1
  While_Iterator/2(ceiling) -> ceiling_He/1
  While_Iterator/1(TTS) -> TTS_He/1
  Palveola/4(fnc_hum_temp) -> While_Iterator/8(fnc_hum_temp)
  Palveola/1(Psw) -> While_Iterator/2(Psw)
  SubS_1/1(bus) -> While_Iterator/5(In1)
  SubS_2/1(bus) -> While_Iterator/6(In2)
  cnc_He/1 -> Palveola/1(Gas concentration), >0/2, While_Iterator/1(cnc_He)
  depth/1 -> Palveola/2("depth, m ")
  Palveola/3(P_alv_INI) -> While_Iterator/7(Palv_INI), SubS_15/3(Palv_INI), SubS_16/3(Palv_INI), SubS_14/3(Palv_INI), SubS_13/3(Palv_INI), SubS_12/3(Palv_INI), SubS_11/3(Palv_INI), SubS_10/3(Palv_INI), SubS_9/3(Palv_INI), SubS_8/3(Palv_INI), SubS_7/3(Palv_INI), SubS_6/3(Palv_INI), SubS_5/3(Palv_INI), SubS_4/3(Palv_INI), SubS_3/3(Palv_INI), SubS_2/3(Palv_INI), SubS_1b/3(Palv_INI), SubS_1/3(Palv_INI)
  Palveola/2(Palv) -> While_Iterator/4(Palv), SubS_1/1(Palv), SubS_15/1(Palv), SubS_16/1(Palv), SubS_14/1(Palv), SubS_13/1(Palv), SubS_12/1(Palv), SubS_11/1(Palv), SubS_10/1(Palv), SubS_9/1(Palv), SubS_8/1(Palv), SubS_7/1(Palv), SubS_6/1(Palv), SubS_5/1(Palv), SubS_4/1(Palv), SubS_3/1(Palv), SubS_2/1(Palv), SubS_1b/1(Palv)
  P_amb_sea_level/1 -> SubS_1/2(Pamb_sea), SubS_15/2(Pamb_sea), SubS_16/2(Pamb_sea), SubS_14/2(Pamb_sea), SubS_13/2(Pamb_sea), SubS_12/2(Pamb_sea), SubS_11/2(Pamb_sea), SubS_10/2(Pamb_sea), SubS_9/2(Pamb_sea), SubS_8/2(Pamb_sea), SubS_7/2(Pamb_sea), SubS_6/2(Pamb_sea), SubS_5/2(Pamb_sea), SubS_4/2(Pamb_sea), SubS_3/2(Pamb_sea), SubS_2/2(Pamb_sea), SubS_1b/2(Pamb_sea)
  zero/1 -> >0/3
  >0/1 -> While_Iterator/3(IC)
  disp_clock/1 -> >0/1
  Half_time_1b/1 -> SubS_1b/4(HT)
  SubS_1b/1(bus) -> While_Iterator/23(In1b)

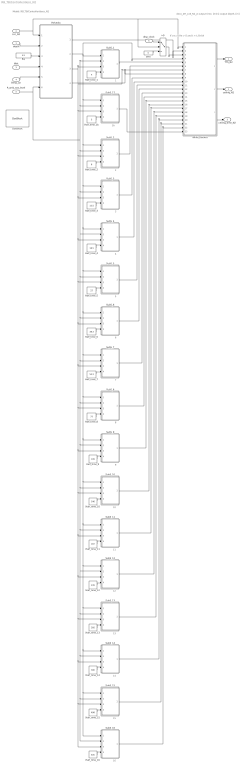
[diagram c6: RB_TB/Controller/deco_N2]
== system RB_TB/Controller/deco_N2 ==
  note: deco_ZH_L16_N2_w output time, [min]; output depth, [m]
  note: 1
  note: 2
  note: 3
  note: 4
  note: 5
  note: 6
  note: 7
  note: 8
  note: 9
  note: 10
  note: 11
  note: 12
  note: 13
  note: 14
  note: 15
  note: 16
  note: Model: RB_TB/Controller/deco_N2
  note: If cnc of He > 0 and t = t_finish
  note: 1b
  depth : Inport  Port=1  LatchInput=off
  cnc_N2 : Inport  Port=2  LatchInput=off
  Wet : Inport  Port=3  LatchInput=off
  Temp_air : Inport  Port=4  LatchInput=off
  P_amb_sea_level : Inport  Port=5  LatchInput=off
  disp_clock : Inport  Port=6  LatchInput=off
  >0 : Switch  Criteria=u2 > Threshold
  DocBlock : simulink/Model-Wide Utilities/DocBlock  DocumentType=Text
  Half_time_1 : Constant  Value=4
  Half_time_10 : Constant  Value=146
  Half_time_11 : Constant  Value=187
  Half_time_12 : Constant  Value=239
  Half_time_13 : Constant  Value=305
  Half_time_14 : Constant  Value=390
  Half_time_15 : Constant  Value=498
  Half_time_16 : Constant  Value=635
  Half_time_1b : Constant  Value=5
  Half_time_2 : Constant  Value=8
  Half_time_3 : Constant  Value=12.5
  Half_time_4 : Constant  Value=18.5
  Half_time_5 : Constant  Value=27
  Half_time_6 : Constant  Value=38.3
  Half_time_7 : Constant  Value=54.3
  Half_time_8 : Constant  Value=77
  Half_time_9 : Constant  Value=109
  Palveola : Subsystem
  RQ : Constant  Value=0.9
  SubS_1 : Subsystem
  SubS_10 : Subsystem
  SubS_11 : Subsystem
  SubS_12 : Subsystem
  SubS_13 : Subsystem
  SubS_14 : Subsystem
  SubS_15 : Subsystem
  SubS_16 : Subsystem
  SubS_17 : Subsystem
  SubS_2 : Subsystem
  SubS_3 : Subsystem
  SubS_4 : Subsystem
  SubS_5 : Subsystem
  SubS_6 : Subsystem
  SubS_7 : Subsystem
  SubS_8 : Subsystem
  SubS_9 : Subsystem
  While_Iterator : Subsystem  TreatAsAtomicUnit=on
  zero : Constant  Value=0
  TTS_N2 : Outport
  ceiling_N2 : Outport  Port=2
  ceiling_time_N2 : Outport  Port=3
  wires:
  P_amb_sea_level/1 -> Palveola/6(P_amb_see_level), SubS_15/2(Pamb_sea), SubS_16/2(Pamb_sea), SubS_14/2(Pamb_sea), SubS_13/2(Pamb_sea), SubS_12/2(Pamb_sea), SubS_11/2(Pamb_sea), SubS_10/2(Pamb_sea), SubS_9/2(Pamb_sea), SubS_8/2(Pamb_sea), SubS_7/2(Pamb_sea), SubS_6/2(Pamb_sea), SubS_5/2(Pamb_sea), SubS_4/2(Pamb_sea), SubS_3/2(Pamb_sea), SubS_2/2(Pamb_sea), SubS_1/2(Pamb_sea), SubS_17/2(Pamb_sea)
  Palveola/2(Palv) -> While_Iterator/4(Palv), SubS_1/1(Palv), SubS_15/1(Palv), SubS_16/1(Palv), SubS_14/1(Palv), SubS_13/1(Palv), SubS_12/1(Palv), SubS_11/1(Palv), SubS_10/1(Palv), SubS_9/1(Palv), SubS_8/1(Palv), SubS_7/1(Palv), SubS_6/1(Palv), SubS_5/1(Palv), SubS_4/1(Palv), SubS_3/1(Palv), SubS_2/1(Palv), SubS_17/1(Palv)
  Palveola/3(P_alv_INI) -> While_Iterator/7(Palv_INI), SubS_15/3(Palv_INI), SubS_16/3(Palv_INI), SubS_14/3(Palv_INI), SubS_13/3(Palv_INI), SubS_12/3(Palv_INI), SubS_11/3(Palv_INI), SubS_10/3(Palv_INI), SubS_9/3(Palv_INI), SubS_8/3(Palv_INI), SubS_7/3(Palv_INI), SubS_6/3(Palv_INI), SubS_5/3(Palv_INI), SubS_4/3(Palv_INI), SubS_3/3(Palv_INI), SubS_2/3(Palv_INI), SubS_17/3(Palv_INI), SubS_1/3(Palv_INI)
  depth/1 -> Palveola/2("depth, m ")
  cnc_N2/1 -> Palveola/1(Gas concentration), While_Iterator/1(cnc_N2), >0/2
  SubS_2/1(bus) -> While_Iterator/6(In2)
  SubS_1/1(bus) -> While_Iterator/5(In1)
  Palveola/1(Psw) -> While_Iterator/2(Psw)
  Palveola/4(fnc_hum_temp) -> While_Iterator/8(fnc_hum_temp)
  While_Iterator/1(TTS) -> TTS_N2/1
  While_Iterator/2(ceiling) -> ceiling_N2/1
  While_Iterator/3(ceiling_time) -> ceiling_time_N2/1
  RQ/1 -> Palveola/3(RQ)
  Wet/1 -> Palveola/4(Humidity)
  Temp_air/1 -> Palveola/5(Temperature)
  SubS_3/1(bus) -> While_Iterator/9(In3)
  SubS_4/1(bus) -> While_Iterator/10(In4)
  SubS_5/1(bus) -> While_Iterator/11(In5)
  SubS_6/1(bus) -> While_Iterator/12(In6)
  SubS_7/1(bus) -> While_Iterator/13(In7)
  SubS_8/1(bus) -> While_Iterator/14(In8)
  SubS_9/1(bus) -> While_Iterator/15(In9)
  SubS_10/1(bus) -> While_Iterator/16(In10)
  SubS_11/1(bus) -> While_Iterator/17(In11)
  SubS_12/1(bus) -> While_Iterator/18(In12)
  SubS_13/1(bus) -> While_Iterator/19(In13)
  SubS_14/1(bus) -> While_Iterator/20(In14)
  SubS_15/1(bus) -> While_Iterator/21(In15)
  SubS_16/1(bus) -> While_Iterator/22(In16)
  Half_time_1/1 -> SubS_1/4(HT)
  Half_time_2/1 -> SubS_2/4(HT)
  Half_time_3/1 -> SubS_3/4(HT)
  Half_time_4/1 -> SubS_4/4(HT)
  Half_time_5/1 -> SubS_5/4(HT)
  Half_time_6/1 -> SubS_6/4(HT)
  Half_time_7/1 -> SubS_7/4(HT)
  Half_time_8/1 -> SubS_8/4(HT)
  Half_time_9/1 -> SubS_9/4(HT)
  Half_time_10/1 -> SubS_10/4(HT)
  Half_time_11/1 -> SubS_11/4(HT)
  Half_time_12/1 -> SubS_12/4(HT)
  Half_time_13/1 -> SubS_13/4(HT)
  Half_time_14/1 -> SubS_14/4(HT)
  Half_time_15/1 -> SubS_15/4(HT)
  Half_time_16/1 -> SubS_16/4(HT)
  disp_clock/1 -> >0/1
  zero/1 -> >0/3
  >0/1 -> While_Iterator/3(IC)
  Half_time_1b/1 -> SubS_17/4(HT)
  SubS_17/1(bus) -> While_Iterator/23(In1b)

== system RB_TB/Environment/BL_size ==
  note: Model: RB_TB/Environment/BL_size
  note: Example: Human dead volume: 3 litre Rebreather dead volume: 5 litre Counterlung residual: 1 litre Counterlung size: 9 litre --------------------------------------------------- From the above BL dead volume: 9 litre Counterlang var volume: 8 litre
  pr_ambient : Inport  Port=1  LatchInput=off
  vol_gas_total : Inport  Port=2  LatchInput=off
  F2 : Fcn  Tag=ee  Priority=306454640  Expr=u(2)+u(1)/2
  Mux1 : Mux  Inputs=2
  Mux2 : Mux  Inputs=2
  Mux5 : Mux  Inputs=2
  PP : Fcn  Tag=ee  Priority=306454640  Expr=u(1)/u(2)
  PP4 : Fcn  Tag=ee  Priority=306454640  Expr=u(1)/u(2)
  Sum2 : Sum  Inputs=++|
  Sum4 : Sum  Inputs=|++
  max_BL_size : Switch  Threshold=16.05
  min_BL_size : Switch  Threshold=7.65
  tidal_volume : Sin  Amplitude=1.4  Frequency=1.4661  SampleTime=0
  vol_cntrlng : Constant  Value=8.4
  vol_dead : Constant  Value=7.65
  BL_size_ini : Outport
  BL_size : Outport  Port=2
  pr_BL : Outport  Port=3
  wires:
  vol_cntrlng/1 -> Sum4/1, Mux2/1
  F2/1 -> BL_size_ini/1
  Sum4/1 -> max_BL_size/1
  min_BL_size/1 -> max_BL_size/3
  vol_dead/1 -> min_BL_size/3, Sum4/2, Mux2/2
  Mux2/1 -> F2/1
  PP/1 -> min_BL_size/1, min_BL_size/2, max_BL_size/2
  Mux5/1 -> PP4/1
  PP4/1 -> pr_BL/1
  Mux1/1 -> PP/1
  pr_ambient/1 -> Mux1/2
  Sum2/1 -> Mux1/1, Mux5/1
  vol_gas_total/1 -> Sum2/2
  tidal_volume/1 -> Sum2/1
  max_BL_size/1 -> BL_size/1, Mux5/2
